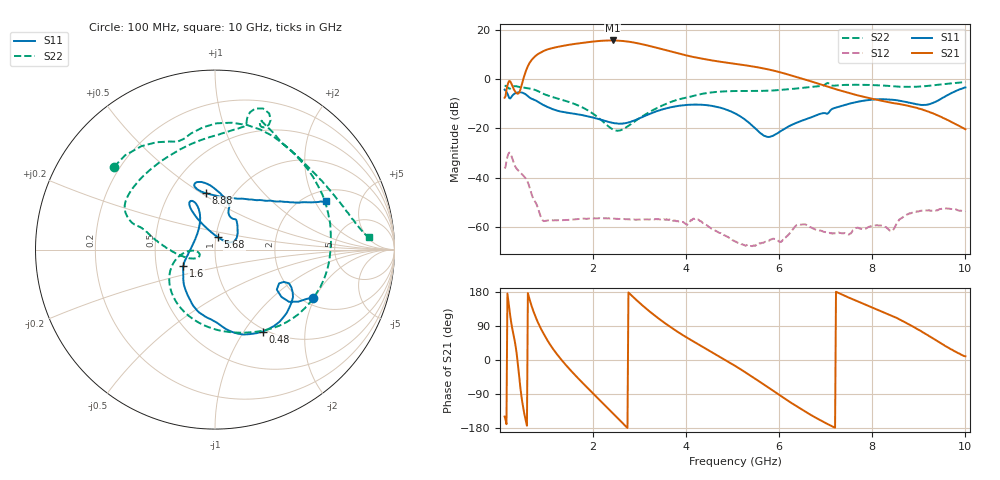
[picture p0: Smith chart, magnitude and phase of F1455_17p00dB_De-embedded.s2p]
! Integrated Device Technology
! Corporate Headquarters
! 6024 Silver Creek Valley Road
! San Jose, CA 95138  USA
! Phone:  1-408-284-8200
! Toll Free:  1-800-223-1366
! Webpage:  http://www.idt.com/
! Timing and RF Division
! 515 Groton Road, Suite 102
! Westford, MA 01886-6024
! Device:  F1455
! Description: 6-bit 0.5 dB Transmit Variable Gain Amplifier
! Frequency:  1400.0 -  2300.00 MHz
! Package:  6x6 mm Thin QFN Plastic Package: 28 pin
! State:  34
! Atten State:  17.0 dB
! Voltage:  +5.00 Volts
! Current:  217.643 mA
! Data:  The device was measured on a the F1455 evaluation board which has
!  individual transmission lines to the RF pins.  Data was collected
!  using a calibrated network analyzer.  The evaluation board was
!  de-embedded using a TRL calibration technique.
!  The reference plane is the edge of the package pin.
!  Pin  1 = CSb
!  Pin  2 = DATA
!  Pin  3 = CLK
!  Pin  4 = RSET
!  Pin  5 = GND
!  Pin  6 = RFIN  = Port 1
!  Pin  7 = GND
!  Pin  8 = NC
!  Pin  9 = NC
!  Pin 10 = NC
!  Pin 11 = NC
!  Pin 12 = NC
!  Pin 13 = NC
!  Pin 14 = /STBY
!  Pin 15 = GND
!  Pin 16 = RFOUT  = Port 2
!  Pin 17 = GND
!  Pin 18 = NC
!  Pin 19 = NC
!  Pin 20 = NC
!  Pin 21 = GND
!  Pin 22 = NC
!  Pin 23 = GND
!  Pin 24 = NC
!  Pin 25 = NC
!  Pin 26 = NC
!  Pin 27 = GND
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# GHz S dB R 50
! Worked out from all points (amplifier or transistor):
!   496 points, 100 MHz to 10 GHz, reference 50 ohm
!   highest |S21| = 15.6 dB at 2.42 GHz (marker M1)
!   |S21| within 3 dB of that: 1.148 GHz to 3.375 GHz (2.227 GHz wide, 98.5 % of centre)
!   unconditionally stable (mu >= 1): start of sweep to end of sweep
!   at 1.74 GHz: K = 57.00, MAG = 15.1 dB, |S12| = -56.7 dB
!   at 5.06 GHz: K = 318.93, MAG = 8.0 dB, |S12| = -66.0 dB
!   at 10 GHz: K = 350.10, MAG = -11.8 dB, |S12| = -53.7 dB
!   S11 on the Smith chart (normalised r, x): 100 MHz: 2.26, -1.92; 480 MHz: 0.96, -1.22; 1.6 GHz: 0.69, -0.13; 5.68 GHz: 1.02, +0.14; 8.88 GHz: 0.75, +0.52; 10 GHz: 2.48, +2.47
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0.1  -4.34 -26.3  -7.60 -149.2  -36.31 46.7  -2.76 140.7
0.26  -6.87 -24.5  -2.53 85.7  -31.99 -76.7  -3.29 95.6
0.38  -5.47 -41.4  -5.98 -4.8  -36.85 -116.0  -3.08 57.6
0.48  -5.53 -59.8  -1.54 -111.3  -38.76 -147.2  -3.41 31.9
0.68  -8.00 -90.9  7.70 142.4  -46.71 142.0  -4.02 -14.7
0.8  -9.03 -106.4  9.88 103.5  -51.48 122.0  -4.77 -41.8
0.94  -10.62 -121.4  11.37 69.0  -57.66 123.5  -6.06 -68.1
1.26  -13.00 -142.2  13.11 9.8  -57.28 99.8  -8.04 -112.2
1.6  -14.10 -153.1  14.22 -38.0  -56.98 70.5  -10.12 -144.6
1.76  -14.62 -157.5  14.64 -58.5  -56.66 59.1  -11.40 -156.4
2.1  -16.16 -168.5  15.37 -100.5  -56.50 39.1  -15.48 -174.7
2.42  -17.76 171.2  15.64 -140.3  -56.65 24.1  -20.40 -171.6
2.8  -17.39 136.1  15.04 173.5  -57.02 11.2  -18.47 -155.9
3.1  -15.10 118.4  13.91 139.9  -56.96 2.1  -14.70 -168.7
3.4  -12.88 112.4  12.50 110.3  -56.82 -7.4  -11.56 178.6
4.1  -10.42 115.7  9.15 53.1  -57.26 -23.5  -7.14 163.2
5.06  -14.02 119.5  6.13 -16.1  -66.00 -60.4  -4.88 148.2
5.68  -23.08 76.3  4.23 -65.6  -66.22 -33.4  -4.80 123.2
6.7  -15.44 41.9  -1.06 -146.4  -60.32 -129.1  -3.20 78.5
8.36  -8.30 107.1  -9.46 119.5  -61.20 133.8  -2.82 62.5
8.88  -9.96 98.9  -11.35 88.0  -53.99 133.6  -3.18 42.1
10  -3.42 23.7  -20.40 9.7  -53.65 50.7  -1.28 4.6
